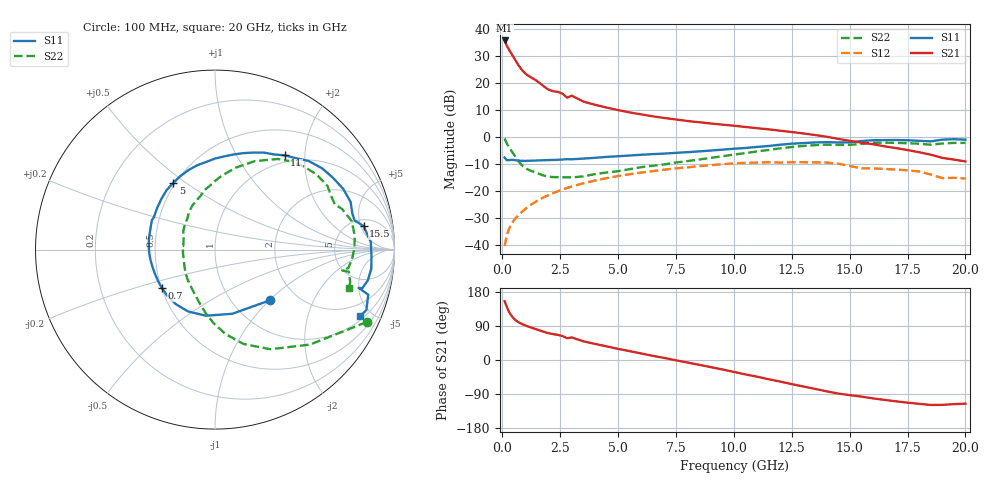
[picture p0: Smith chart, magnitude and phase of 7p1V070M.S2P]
! Infineon Technologies  Discrete & RF Semiconductors
! bfp620
! VCE =  1.0 V,  IC =  70 mA
! Common Emitter S-Parameters:  Sep 2002
# GHz  S  MA  R  50
!  f  S11  S21  S12  S22
! GHz  MAG  ANG  MAG  ANG  MAG  ANG  MAG  ANG
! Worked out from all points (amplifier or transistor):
!   59 points, 100 MHz to 20 GHz, reference 50 ohm
!   highest |S21| = 35.7 dB at 100 MHz (marker M1)
!   |S21| within 3 dB of that: start of sweep to 265 MHz
!   unconditionally stable (mu >= 1): 1.914 GHz to 2.296 GHz; 3.141 GHz to 10.28 GHz; 17.05 GHz to end of sweep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
!   at 1 GHz: K = 0.90, MSG = 25.0 dB, |S12| = -26.6 dB
!   at 5.5 GHz: K = 1.04, MAG = 10.2 dB, |S12| = -13.8 dB
!   at 20 GHz: K = 1.41, MAG = -0.6 dB, |S12| = -15.4 dB
!   S11 on the Smith chart (normalised r, x): 100 MHz: 1.47, -1.01; 700 MHz: 0.50, -0.25; 5 GHz: 0.49, +0.45; 11 GHz: 0.88, +1.61; 15.5 GHz: 6.35, +5.60; 20 GHz: 1.20, -4.27
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0.1  0.4162 -42.8  61.09 155.5  0.0095 79.1  0.9369 -25.5
0.2  0.3703 -74.9  48.62 139.2  0.0154 68.1  0.7483 -45.0
0.3  0.372 -97.8  40.61 126.1  0.0204 64.5  0.6354 -60.9
0.4  0.3759 -113.8  34.46 116.4  0.0247 63.0  0.5492 -73.2
0.5  0.3743 -126.1  29.27 109.2  0.0285 62.3  0.4743 -82.9
0.6  0.3698 -136.1  24.87 103.9  0.0322 62.1  0.4094 -91.2
0.7  0.3653 -144.4  21.27 99.7  0.0357 62.0  0.356 -98.6
0.8  0.3622 -151.3  18.46 96.4  0.0393 61.9  0.3149 -105.3
1  0.3606 -161.3  14.88 91.1  0.0466 61.7  0.2646 -116.6
1.4  0.3652 -174.0  11.54 82.4  0.0615 60.4  0.223 -133.9
1.9  0.3718 172.1  7.976 72.4  0.0802 57.1  0.1872 -157.1
2.8  0.3881 154.9  5.329 57.4  0.1136 49.3  0.1792 173.3
3  0.3853 152.5  5.812 59.5  0.1209 47.4  0.178 173.5
3.5  0.3974 144.1  4.514 49.2  0.1388 42.4  0.1857 160.3
5  0.4391 121.9  3.141 29.4  0.1887 26.9  0.2321 131.4
7  0.4913 95.5  2.242 5.4  0.2476 6.3  0.3095 105.1
10.5  0.6243 58.1  1.53 -38.0  0.3313 -34.2  0.5013 70.8
11  0.6531 53.6  1.452 -44.0  0.3348 -39.9  0.5389 66.0
13.5  0.7903 25.4  1.086 -76.1  0.3378 -70.1  0.7041 36.3
15.5  0.8382 9.0  0.787 -96.5  0.2624 -92.2  0.7434 17.7
17  0.8772 -6.9  0.622 -109.0  0.2488 -101.3  0.7767 0.5
20  0.8897 -24.6  0.352 -115.2  0.1694 -111.7  0.7757 -16.2
